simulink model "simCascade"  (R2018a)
settings: Solver=ode15s  StartTime=0.0  StopTime=tsim  MaxStep=0.1  RelTol=1e-3
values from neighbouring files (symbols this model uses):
  d_step = dnom + dnom.*[0;0]    [runCascade.m]    (also in Main.m = [Fh, Tcin, Thin]; Main_OL.m = [Fh, Tcin+0, Thin]; runTestCalcBlk.m = [Fh, Tcin, Thin])
  dnom = zeros(2,1)    [PI_Tank.m]    (also in runCascade.m)
  Kc = 0    [PI_Tank.m]    (also in runCascade.m = tauQ/(tauC+theta); runTransformedMVs.m = 0.01; Main.m = 1/k*tau/(tauC+theta); runTransf.m = 1/kM(i)*tau(i)/(tauCM(i)+theta(i)))
  KIS = 1/0.024*1/1    (= 41.6666666667)    [runCascade.m]    (also in runTransformedMVs.m)
  p = [V;rho;cp;qnom;MV;transf]    [PI_Tank.m]    (also in runCascade.m = [V;rho;cp;A;tau0;MV;transf]; runTransformedMVs.m = [V;rho;cp;A;tau0;MV;transf]; Main.m = [N, Fc0, rhoc, rhoh,U,A,cpc,cph]; Main_OL.m = [N, Fc0, rhoc, rhoh,U,A,cpc,cph])
  tauI = 1    [PI_Tank.m]    (also in runCascade.m = min(tauQ,4*(tauC+theta)); runTransformedMVs.m = 400; Main.m = min(tau,4*(tauC+theta)); runTransf.m = min(tau(i), 4*(tauCM(i)+theta(i))))
  Tnom = 50    [PI_Tank.m]    (also in runCascade.m; runTransformedMVs.m)
  Tstep = Tnom+10    (= 60)    [PI_Tank.m]    (also in runCascade.m = 40; runTransformedMVs.m = -10)
  tstep_d = 10    [PI_Tank.m]    (also in runCascade.m)
  tstep_T = 50    [PI_Tank.m]    (also in runCascade.m = 500)
  ubias = Qnom    (= 167.2)    [PI_Tank.m]    (also in runCascade.m = 1672; runTransformedMVs.m = 1672)
  umax = inf    [runCascade.m]    (also in runTransformedMVs.m = 5016)
  vbias = Tnom    (= 50)    [runCascade.m]    (also in runTransformedMVs.m = 0)
undefined symbols (not defined in the file or in its folder): CalcBlock_cascade, Tank

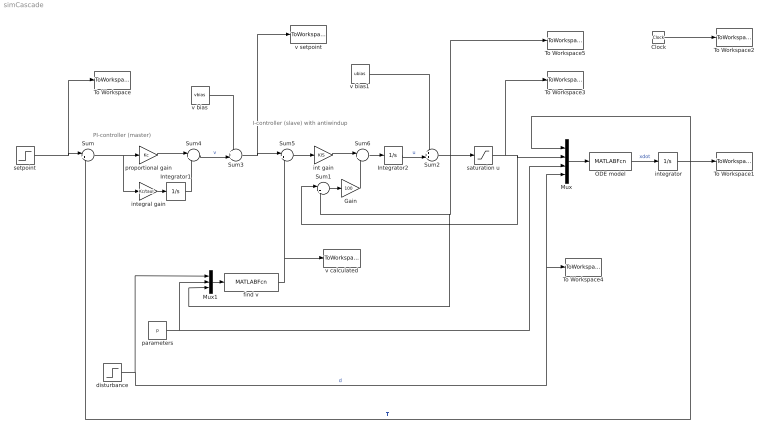
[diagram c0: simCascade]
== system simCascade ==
  note: PI-controller (master)
  note: I-controller (slave) with antiwindup
  " integrator" : Integrator  InitialCondition=Tnom
  Clock : Clock
  Gain : Gain  Gain=100  Multiplication=Matrix(K*u)
  Integrator1 : Integrator
  Integrator2 : Integrator
  Mux : Mux
  Mux1 : Mux  Inputs=3
  ODE model : MATLABFcn  MATLABFcn=Tank(u(1), u(2),u(3:9),u(10:11))  OutputDimensions=1
  Sum : Sum  Inputs=|+-
  Sum1 : Sum  Inputs=|+-
  Sum2 : Sum  Inputs=++|
  Sum3 : Sum  Inputs=++|
  Sum4 : Sum  Inputs=|++
  Sum5 : Sum  Inputs=|+-
  Sum6 : Sum  Inputs=|++
  To Workspace : ToWorkspace  VariableName=Tsp  SampleTime=-1
  To Workspace1 : ToWorkspace  VariableName=T  SampleTime=-1
  To Workspace2 : ToWorkspace  VariableName=time  SampleTime=-1
  To Workspace3 : ToWorkspace  VariableName=u  SampleTime=-1
  To Workspace4 : ToWorkspace  VariableName=d  SampleTime=-1
  To Workspace5 : ToWorkspace  VariableName=uc  SampleTime=-1
  disturbance : Step  Time=tstep_d  Before=dnom  After=d_step  SampleTime=0
  find v : MATLABFcn  MATLABFcn=CalcBlock_cascade(u(1:2),u(3:9),u(10))  OutputDimensions=1
  int gain : Gain  Gain=KIS  Multiplication=Matrix(K*u)
  integral gain : Gain  Gain=Kc/tauI  Multiplication=Matrix(K*u)
  parameters : Constant  Value=p
  proportional gain : Gain  Gain=Kc  Multiplication=Matrix(K*u)
  saturation u : Saturate  UpperLimit=umax  LowerLimit=0
  setpoint : Step  Time=tstep_T  Before=Tnom  After=Tstep  SampleTime=0
  v bias : Constant  Value=vbias
  v bias1 : Constant  Value=ubias
  v calculated : ToWorkspace  VariableName=vc  SampleTime=-1
  v setpoint : ToWorkspace  VariableName=v  SampleTime=-1
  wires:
  " integrator"/1 -> Mux/1, To Workspace1/1, Sum/2  "T"
  Mux/1 -> ODE model/1
  Clock/1 -> To Workspace2/1
  Sum/1 -> integral gain/1, proportional gain/1
  Sum4/1 -> Sum3/2  "v"
  ODE model/1 -> " integrator"/1  "xdot"
  integral gain/1 -> Integrator1/1
  proportional gain/1 -> Sum4/1
  Integrator1/1 -> Sum4/2
  disturbance/1 -> Mux/4, To Workspace4/1, Mux1/1  "d"
  parameters/1 -> Mux1/2, Mux/3
  v bias/1 -> Sum3/1
  setpoint/1 -> To Workspace/1, Sum/1
  find v/1 -> v calculated/1, Sum5/2
  int gain/1 -> Sum6/1
  Sum5/1 -> int gain/1
  Integrator2/1 -> Sum2/2  "u"
  Sum2/1 -> Mux1/3, Sum1/2, To Workspace5/1, saturation u/1
  Mux1/1 -> find v/1
  saturation u/1 -> To Workspace3/1, Sum1/1, Mux/2
  Sum3/1 -> Sum5/1, v setpoint/1
  v bias1/1 -> Sum2/1
  Sum6/1 -> Integrator2/1
  Gain/1 -> Sum6/2
  Sum1/1 -> Gain/1
